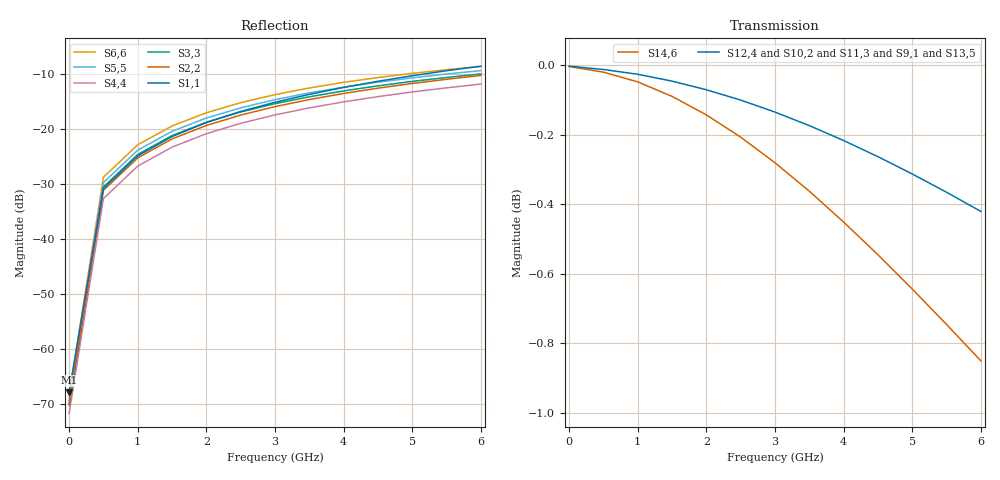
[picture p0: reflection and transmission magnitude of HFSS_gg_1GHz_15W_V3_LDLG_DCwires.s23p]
! Touchstone file from project HFSS_gg_1GHz_15W_V3_LDLG_DCwires
! Exported from HFSS 15.0.0
# GHZ S MA R 50.000000
! Terminal data exported
! Port[1] = 1LeadDC3_T1
! Port[2] = 2LeadDC2_T1
! Port[3] = 3LeadDC1_T1
! Port[4] = 4LeadRF_T1
! Port[5] = 5LeadDC1b_T1
! Port[6] = 6LeadDC2b_T1
! Port[7] = 7LeadDC3b_T1
! Port[8] = LeadOUT_T1
! Port[9] = Rectangle38_T1
! Port[10] = Rectangle37_T1
! Port[11] = Rectangle16_2_T1
! Port[12] = Rectangle36_T1
! Port[13] = Rectangle14_2_T1
! Port[14] = Rectangle17_T1
! Port[15] = Rectangle18_T1
! Port[16] = Rectangle26_T1
! Port[17] = Rectangle27_T1
! Port[18] = Rectangle28_3_T1
! Port[19] = Rectangle29_T1
! Port[20] = Rectangle30_T1
! Port[21] = Rectangle31_T1
! Port[22] = Rectangle32_T1
! Port[23] = Rectangle33_T1
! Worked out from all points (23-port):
!   13 points, 1 MHz to 6 GHz, reference 50 ohm
!   strongest paths, dB at 1 MHz, 1.501 GHz, 3.001 GHz, 4.501 GHz, 6 GHz:
!     S12,4: 0.0, 0.0, -0.1, -0.3, -0.4
!     S10,2: 0.0, -0.1, -0.2, -0.4, -0.6
!     S11,3: 0.0, -0.1, -0.2, -0.4, -0.6
!     S9,1: 0.0, -0.1, -0.2, -0.4, -0.8
!     S13,5: 0.0, -0.1, -0.2, -0.5, -0.7
!     S14,6: 0.0, -0.1, -0.3, -0.5, -0.9
!   lowest |S11| = -67.8 dB at 1 MHz (marker M1), VSWR 1.00, Z = 50 + j0.00638 ohm
!   |S11| at or under -10 dB: start of sweep to 5.194 GHz
